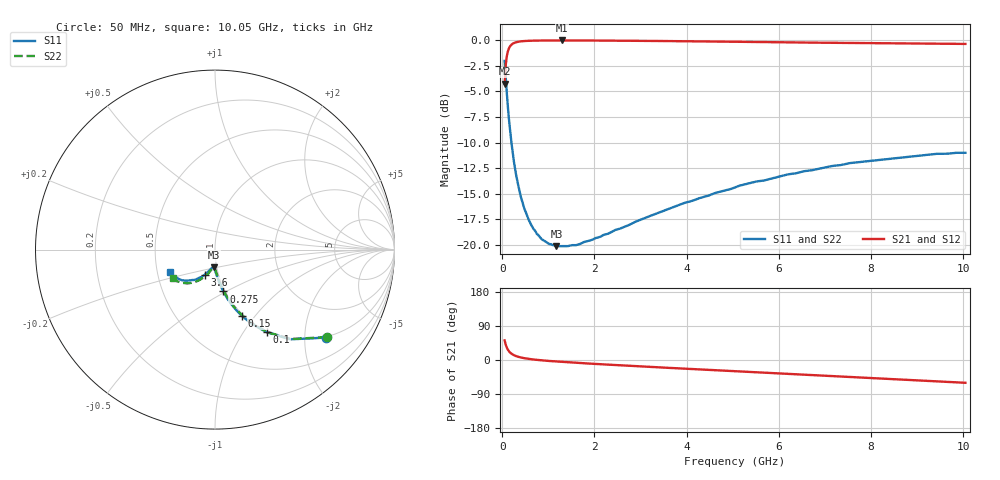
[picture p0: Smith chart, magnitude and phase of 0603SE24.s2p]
! AVX Thin Film Operation		Date: August 2001
! Description: Accu-P® Series, Thin Film, SMD, RF Capacitor
! Part Number: 06033J240FBT
! 50 MHz  -  10.05 GHz
! Serial Measurements
# mhz S db R 50
!	S11		S21		S12		S22
!	dB	Phase	dB	Phase	dB	Phase	dB	Phase
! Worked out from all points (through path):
!   401 points, 50 MHz to 10.05 GHz, reference 50 ohm
!   highest |S21| = -0.05 dB at 1.3 GHz (marker M1); lowest = -4.3 dB at 50 MHz (marker M2)
!   group delay of S21, straight-line fit = 18.8 ps
!   lowest |S11| = -20.1 dB at 1.175 GHz (marker M3), VSWR 1.22, Z = 48.3 - j9.6 ohm
!   |S11| at or under -10 dB: 198.1 MHz to end of sweep
!   |S22| runs from -20.1 to -2.0 dB; largest |S21 - S12| = 0
!   S11 on the Smith chart (normalised r, x): 50 MHz: 0.98, -2.55; 100 MHz: 0.98, -1.28; 150 MHz: 0.98, -0.86; 275 MHz: 0.98, -0.48; 3.6 GHz: 0.86, -0.24; 10.05 GHz: 0.58, -0.16
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50  -2.04 -38.3  -4.26 51.8  -4.26 51.8  -2.04 -38.1
100  -5.29 -57.9  -1.52 32.2  -1.52 32.2  -5.29 -57.7
125  -6.73 -63.7  -1.04 26.4  -1.04 26.4  -6.73 -63.3
150  -8.00 -67.9  -0.76 22.2  -0.76 22.2  -8.00 -67.5
175  -9.08 -71.1  -0.58 19.1  -0.58 19.1  -9.08 -70.5
200  -10.07 -73.6  -0.45 16.6  -0.45 16.6  -10.07 -73.0
275  -12.48 -78.8  -0.26 11.5  -0.26 11.5  -12.48 -78.0
350  -14.26 -82.1  -0.17 8.3  -0.17 8.3  -14.26 -81.1
425  -15.62 -84.4  -0.12 6.0  -0.12 6.0  -15.62 -83.2
525  -16.97 -86.7  -0.09 3.8  -0.09 3.8  -16.97 -85.3
625  -18.01 -88.4  -0.07 2.1  -0.07 2.1  -18.01 -86.9
875  -19.48 -91.8  -0.05 -1.1  -0.05 -1.1  -19.48 -89.8
1175  -20.10 -94.7  -0.05 -4.0  -0.05 -4.0  -20.10 -92.5
1300  -20.10 -95.8  -0.05 -5.0  -0.05 -5.0  -20.10 -93.5
1725  -19.80 -99.2  -0.05 -8.3  -0.05 -8.3  -19.80 -96.6
3400  -16.83 -110.9  -0.10 -19.4  -0.10 -19.4  -16.83 -106.9
3600  -16.48 -112.1  -0.11 -20.7  -0.11 -20.7  -16.48 -109.1
5050  -14.38 -121.4  -0.17 -29.7  -0.17 -29.7  -14.32 -117.4
6725  -12.70 -132.0  -0.26 -39.9  -0.26 -39.9  -12.60 -127.0
7575  -11.99 -137.2  -0.30 -45.1  -0.30 -45.1  -11.99 -132.1
8400  -11.59 -143.1  -0.34 -50.2  -0.34 -50.2  -11.49 -137.1
10050  -11.00 -153.6  -0.39 -60.1  -0.39 -60.1  -10.92 -145.8
